| TEXAS INSTRUMENTS INCORPORATED
| Standard Linear and Logic Group
| IBIS Model of SN74ALVC164245
| 16-BIT 2.5-V TO 3.3-V/3.3-V TO 5-V LEVEL-SHIFTING TRANSCEIVER WITH
| 3-STATE OUTPUTS
| This file contains package information for the following:
|  TSSOP 48-pin (DGG) package as [Component] ALVC164245_DGG
|  SSOP 48-pin (DL) package as [Component] ALVC164245_DL
|  VFBGA 48-pin (GQL) package as [Component] ALVC164245_GQL
|  VFBGA 48-pin (ZQL) package as [Component] ALVC164245_ZQL
| This device can be powered at the following Vccs:
|  2.5 volt Vcc
|  3.3 volt Vcc
|  5.0 volt Vcc
| This file provides unique models under the [Model Selector] for each Vcc.
| For operation at a specific Vcc, select the appropriate model after each
| [Model Selector] keyword.
[IBIS Ver]   3.2
[Comment char]  |_char
[File Name]   sn74alvc164245.ibs
[File Rev]   1.1 | b_die
[Date]   September 14, 2004
[Source]   Data created from TI-SPICE simulations at TI-SLL.
[Notes]   The following is an IBIS list for the ALVC164245.
   Please contact sllibis@ti.com with questions and
   comments concerning SLL IBIS models.
   This IBIS model is created from a BA (back annotated
   netlist)
   - FILE REV HISTORY
   - 1.1 Release IBIS file on 09/29/04
   - Power clamp data has been deleted from DIR and NOE models
   since there is no power clamp diode for those inputs.
[Disclaimer] Property of Texas Instruments Incorporated.  Unauthorized
   reproduction and/or distribution is strictly prohibited.
   This product is protected under copyright law.
   Created  2004, (C) Copyright  2004, Texas Instruments
   Incorporated, All Rights Reserved
   UNLESS THERE IS A SIGNED, WRITTEN AGREEMENT TO THE
   CONTRARY, TEXAS INSTRUMENTS (TI) IS PROVIDING THE IBIS
   MODELS  AND WITHOUT ANY WARRANTY, EXPRESSED OR
   IMPLIED.  TI assumes no liability for:
   1) the accuracy of the IBIS models provided to your
   company;
   2) the proper functioning of these IBIS Models in your
   design or for any resulting applications; or
   3) infringement of patents, copyrights or intellectual
   property rights resulting from your use of these IBIS
   models.
   TI provides IBIS Models as a service to our customers.
   You and your company shall not distribute, sell or give
   these models to anyone else without prior written
   permission from TI.
   TI reserves the right to make changes to our products or
   to discontinue any semiconductor product or service
   without notice, and advises our customers to obtain the
   latest version of relevant information to verify, before
   placing orders, that the information being relied on is
   current.
   Please be aware that your receipt and use of the IBIS
   information provided shall serve as acceptance of these
   terms and conditions.  If you do not accept these terms,
   you should return or destroy the IBIS models and any
   other accompanying information immediately.
| Component ALVC164245_DGG 48-pin TSSOP
[Component]   ALVC164245_DGG
[Manufacturer]   Texas Instruments, Inc.
[Package]
|   typ   min   max
R_pkg   4.400e-02   3.800e-02   5.100e-02
L_pkg   3.019e-09   2.486e-09   4.099e-09
C_pkg   5.070e-13   3.340e-13   8.090e-13
[Pin]   signal_name   model_name   R_pin   L_pin   C_pin
1   1DIR   ALVC164245_DIR   4.100e-02   4.017e-09   7.590e-13
2   1B1   ALVC164245_BIO   4.200e-02   3.737e-09   7.920e-13
3   1B2   ALVC164245_BIO   4.200e-02   3.480e-09   6.610e-13
4   GND   GND   3.800e-02   3.131e-09   5.750e-13
5   1B3   ALVC164245_BIO   4.700e-02   3.122e-09   5.660e-13
6   1B4   ALVC164245_BIO   4.300e-02   2.948e-09   5.040e-13
7   VCCB   POWER   4.500e-02   2.845e-09   3.970e-13
8   1B5   ALVC164245_BIO   4.900e-02   2.835e-09   3.940e-13
9   1B6   ALVC164245_BIO   4.800e-02   2.715e-09   3.780e-13
10   GND   GND   5.000e-02   2.664e-09   3.630e-13
11   1B7   ALVC164245_BIO   5.000e-02   2.585e-09   3.480e-13
12   1B8   ALVC164245_BIO   4.900e-02   2.550e-09   3.370e-13
13   2B1   ALVC164245_BIO   4.900e-02   2.541e-09   3.360e-13
14   2B2   ALVC164245_BIO   5.000e-02   2.574e-09   3.480e-13
15   GND   GND   4.900e-02   2.618e-09   3.590e-13
16   2B3   ALVC164245_BIO   4.600e-02   2.671e-09   3.750e-13
17   2B4   ALVC164245_BIO   4.500e-02   2.754e-09   3.890e-13
18   VCCB   POWER   4.400e-02   2.823e-09   4.500e-13
19   2B5   ALVC164245_BIO   4.200e-02   2.968e-09   5.030e-13
20   2B6   ALVC164245_BIO   5.100e-02   3.108e-09   5.350e-13
21   GND   GND   4.200e-02   3.175e-09   5.870e-13
22   2B7   ALVC164245_BIO   4.100e-02   3.449e-09   6.780e-13
23   2B8   ALVC164245_BIO   4.400e-02   3.766e-09   8.040e-13
24   2DIR   ALVC164245_DIR   4.300e-02   4.065e-09   7.610e-13
25   2NOE   ALVC164245_NOE   4.100e-02   3.994e-09   7.570e-13
26   2A8   ALVC164245_AIO   3.900e-02   3.649e-09   7.890e-13
27   2A7   ALVC164245_AIO   3.800e-02   3.362e-09   6.600e-13
28   GND   GND   3.800e-02   3.082e-09   5.740e-13
29   2A6   ALVC164245_AIO   4.400e-02   2.990e-09   5.220e-13
30   2A5   ALVC164245_AIO   4.100e-02   2.917e-09   4.950e-13
31   VCCA   POWER   4.300e-02   2.820e-09   4.480e-13
32   2A4   ALVC164245_AIO   4.300e-02   2.699e-09   3.850e-13
33   2A3   ALVC164245_AIO   4.500e-02   2.628e-09   3.720e-13
34   GND   GND   4.600e-02   2.556e-09   3.560e-13
35   2A2   ALVC164245_AIO   4.600e-02   2.495e-09   3.440e-13
36   2A1   ALVC164245_AIO   4.700e-02   2.487e-09   3.340e-13
37   1A8   ALVC164245_AIO   4.700e-02   2.490e-09   3.350e-13
38   1A7   ALVC164245_AIO   4.600e-02   2.486e-09   3.430e-13
39   GND   GND   4.500e-02   2.566e-09   3.560e-13
40   1A6   ALVC164245_AIO   4.400e-02   2.639e-09   3.740e-13
41   1A5   ALVC164245_AIO   4.300e-02   2.701e-09   3.860e-13
42   VCCA   POWER   4.300e-02   2.817e-09   4.500e-13
43   1A4   ALVC164245_AIO   4.100e-02   2.935e-09   5.010e-13
44   1A3   ALVC164245_AIO   4.700e-02   3.035e-09   5.290e-13
45   GND   GND   4.300e-02   3.171e-09   5.890e-13
46   1A2   ALVC164245_AIO   4.000e-02   3.415e-09   6.820e-13
47   1A1   ALVC164245_AIO   4.300e-02   3.741e-09   8.090e-13
48   1NOE   ALVC164245_NOE   4.400e-02   4.099e-09   7.640e-13
| Component ALVC164245_DL 48-pin SSOP
[Component]   ALVC164245_DL
[Manufacturer]   Texas Instruments, Inc.
[Package]
|   typ   min   max
R_pkg   4.800e-02   3.800e-02   5.300e-02
L_pkg   6.046e-09   5.084e-09   7.968e-09
C_pkg   8.130e-13   5.690e-13   1.157e-12
[Pin]   signal_name   model_name   R_pin   L_pin   C_pin
1   1DIR   ALVC164245_DIR   4.600e-02   7.968e-09   1.017e-12
2   1B1   ALVC164245_BIO   4.400e-02   7.299e-09   1.157e-12
3   1B2   ALVC164245_BIO   4.300e-02   6.765e-09   1.058e-12
4   GND   GND   4.100e-02   6.269e-09   9.330e-13
5   1B3   ALVC164245_BIO   3.800e-02   5.856e-09   8.290e-13
6   1B4   ALVC164245_BIO   4.600e-02   5.802e-09   7.900e-13
7   VCCB   POWER   5.000e-02   5.656e-09   7.380e-13
8   1B5   ALVC164245_BIO   5.300e-02   5.500e-09   6.430e-13
9   1B6   ALVC164245_BIO   5.200e-02   5.304e-09   6.060e-13
10   GND   GND   5.300e-02   5.189e-09   5.830e-13
11   1B7   ALVC164245_BIO   5.100e-02   5.084e-09   5.690e-13
12   1B8   ALVC164245_BIO   5.300e-02   5.862e-09   8.330e-13
13   2B1   ALVC164245_BIO   5.300e-02   5.862e-09   8.330e-13
14   2B2   ALVC164245_BIO   5.100e-02   5.084e-09   5.690e-13
15   GND   GND   5.300e-02   5.189e-09   5.830e-13
16   2B3   ALVC164245_BIO   5.200e-02   5.304e-09   6.060e-13
17   2B4   ALVC164245_BIO   5.300e-02   5.500e-09   6.430e-13
18   VCCB   POWER   5.000e-02   5.656e-09   7.380e-13
19   2B5   ALVC164245_BIO   4.600e-02   5.802e-09   7.900e-13
20   2B6   ALVC164245_BIO   3.800e-02   5.856e-09   8.290e-13
21   GND   GND   4.100e-02   6.269e-09   9.330e-13
22   2B7   ALVC164245_BIO   4.300e-02   6.765e-09   1.058e-12
23   2B8   ALVC164245_BIO   4.400e-02   7.299e-09   1.157e-12
24   2DIR   ALVC164245_DIR   4.600e-02   7.968e-09   1.017e-12
25   2NOE   ALVC164245_NOE   4.600e-02   7.968e-09   1.017e-12
26   2A8   ALVC164245_AIO   4.400e-02   7.299e-09   1.157e-12
27   2A7   ALVC164245_AIO   4.300e-02   6.765e-09   1.058e-12
28   GND   GND   4.100e-02   6.269e-09   9.330e-13
29   2A6   ALVC164245_AIO   3.800e-02   5.856e-09   8.290e-13
30   2A5   ALVC164245_AIO   4.600e-02   5.802e-09   7.900e-13
31   VCCA   POWER   5.000e-02   5.656e-09   7.380e-13
32   2A4   ALVC164245_AIO   5.300e-02   5.500e-09   6.430e-13
33   2A3   ALVC164245_AIO   5.200e-02   5.304e-09   6.060e-13
34   GND   GND   5.300e-02   5.189e-09   5.830e-13
35   2A2   ALVC164245_AIO   5.100e-02   5.084e-09   5.690e-13
36   2A1   ALVC164245_AIO   5.300e-02   5.862e-09   8.330e-13
37   1A8   ALVC164245_AIO   5.300e-02   5.862e-09   8.330e-13
38   1A7   ALVC164245_AIO   5.100e-02   5.084e-09   5.690e-13
39   GND   GND   5.300e-02   5.189e-09   5.830e-13
40   1A6   ALVC164245_AIO   5.200e-02   5.304e-09   6.060e-13
41   1A5   ALVC164245_AIO   5.300e-02   5.500e-09   6.430e-13
42   VCCA   POWER   5.000e-02   5.656e-09   7.380e-13
43   1A4   ALVC164245_AIO   4.600e-02   5.802e-09   7.900e-13
44   1A3   ALVC164245_AIO   3.800e-02   5.856e-09   8.290e-13
45   GND   GND   4.100e-02   6.269e-09   9.330e-13
46   1A2   ALVC164245_AIO   4.300e-02   6.765e-09   1.058e-12
47   1A1   ALVC164245_AIO   4.400e-02   7.299e-09   1.157e-12
48   1NOE   ALVC164245_NOE   4.600e-02   7.967e-09   1.017e-12
| Component ALVC164245_GQL 48-pin VFBGA
[Component]   ALVC164245_GQL
[Manufacturer]   Texas Instruments, Inc.
[Package]
|   typ   min   max
R_pkg   7.900e-02   4.500e-02   9.400e-02
L_pkg   2.264e-09   1.398e-09   2.722e-09
C_pkg   3.060e-13   1.170e-13   4.040e-13
[Pin]   signal_name   model_name   R_pin   L_pin   C_pin
A1   1DIR   ALVC164245_DIR   5.10E-02   1.53E-09   2.10E-13
B2   1B1   ALVC164245_BIO   7.30E-02   2.57E-09   3.12E-13
B1   1B2   ALVC164245_BIO   7.10E-02   1.84E-09   2.32E-13
B3   GND   GND   9.40E-02   2.72E-09   3.83E-13
C2   1B3   ALVC164245_BIO   8.90E-02   2.53E-09   3.50E-13
C1   1B4   ALVC164245_BIO   7.10E-02   1.83E-09   2.31E-13
C3   VCCB   POWER   9.40E-02   2.72E-09   3.92E-13
D2   1B5   ALVC164245_BIO   9.00E-02   2.55E-09   3.52E-13
D1   1B6   ALVC164245_BIO   7.20E-02   1.85E-09   2.44E-13
D3   GND   GND   9.40E-02   2.72E-09   4.03E-13
E2   1B7   ALVC164245_BIO   8.90E-02   2.54E-09   3.51E-13
E1   1B8   ALVC164245_BIO   7.20E-02   1.85E-09   2.27E-13
F1   2B1   ALVC164245_BIO   7.20E-02   1.85E-09   2.27E-13
F2   2B2   ALVC164245_BIO   8.90E-02   2.54E-09   3.51E-13
G3   GND   GND   9.40E-02   2.72E-09   4.04E-13
G1   2B3   ALVC164245_BIO   7.20E-02   1.85E-09   2.44E-13
G2   2B4   ALVC164245_BIO   9.00E-02   2.55E-09   3.52E-13
H3   VCCB   POWER   9.40E-02   2.72E-09   3.92E-13
H1   2B5   ALVC164245_BIO   7.00E-02   1.83E-09   2.31E-13
H2   2B6   ALVC164245_BIO   8.80E-02   2.52E-09   3.50E-13
J3   GND   GND   9.30E-02   2.71E-09   3.82E-13
J1   2B7   ALVC164245_BIO   7.10E-02   1.85E-09   2.33E-13
J2   2B8   ALVC164245_BIO   5.60E-02   2.61E-09   3.90E-13
K1   2DIR   ALVC164245_DIR   4.50E-02   1.40E-09   1.17E-13
K6   2NOE   ALVC164245_NOE   4.50E-02   1.51E-09   1.93E-13
J5   2A8   ALVC164245_AIO   5.50E-02   2.49E-09   3.13E-13
J6   2A7   ALVC164245_AIO   7.00E-02   1.82E-09   2.30E-13
J4   GND   GND   9.30E-02   2.70E-09   3.82E-13
H5   2A6   ALVC164245_AIO   8.90E-02   2.53E-09   3.50E-13
H6   2A5   ALVC164245_AIO   7.10E-02   1.83E-09   2.30E-13
H4   VCCA   POWER   9.40E-02   2.72E-09   3.91E-13
G5   2A4   ALVC164245_AIO   9.00E-02   2.55E-09   3.52E-13
G6   2A3   ALVC164245_AIO   7.20E-02   1.85E-09   2.44E-13
G4   GND   GND   9.40E-02   2.72E-09   4.04E-13
F5   2A2   ALVC164245_AIO   8.80E-02   2.51E-09   3.49E-13
F6   2A1   ALVC164245_AIO   7.20E-02   1.85E-09   2.27E-13
E6   1A8   ALVC164245_AIO   7.10E-02   1.85E-09   2.27E-13
E5   1A7   ALVC164245_AIO   8.90E-02   2.53E-09   3.50E-13
D4   GND   GND   9.40E-02   2.72E-09   4.03E-13
D6   1A6   ALVC164245_AIO   7.20E-02   1.85E-09   2.43E-13
D5   1A5   ALVC164245_AIO   8.90E-02   2.55E-09   3.52E-13
C4   VCCA   POWER   9.40E-02   2.72E-09   3.91E-13
C6   1A4   ALVC164245_AIO   7.10E-02   1.83E-09   2.30E-13
C5   1A3   ALVC164245_AIO   8.90E-02   2.54E-09   3.50E-13
B4   GND   GND   9.30E-02   2.71E-09   3.82E-13
B6   1A2   ALVC164245_AIO   7.10E-02   1.83E-09   2.27E-13
B5   1A1   ALVC164245_AIO   7.30E-02   2.69E-09   3.80E-13
A6   1NOE   ALVC164245_NOE   5.10E-02   1.42E-09   1.33E-13
| Component ALVC164245_ZQL 48-pin VFBGA
[Component]   ALVC164245_ZQL
[Manufacturer]   Texas Instruments, Inc.
[Package]
|   typ   min   max
R_pkg   7.900e-02   4.500e-02   9.400e-02
L_pkg   2.264e-09   1.398e-09   2.722e-09
C_pkg   3.060e-13   1.170e-13   4.040e-13
[Pin]   signal_name   model_name   R_pin   L_pin   C_pin
A1   1DIR   ALVC164245_DIR   5.10E-02   1.53E-09   2.10E-13
B2   1B1   ALVC164245_BIO   7.30E-02   2.57E-09   3.12E-13
B1   1B2   ALVC164245_BIO   7.10E-02   1.84E-09   2.32E-13
B3   GND   GND   9.40E-02   2.72E-09   3.83E-13
C2   1B3   ALVC164245_BIO   8.90E-02   2.53E-09   3.50E-13
C1   1B4   ALVC164245_BIO   7.10E-02   1.83E-09   2.31E-13
C3   VCCB   POWER   9.40E-02   2.72E-09   3.92E-13
D2   1B5   ALVC164245_BIO   9.00E-02   2.55E-09   3.52E-13
D1   1B6   ALVC164245_BIO   7.20E-02   1.85E-09   2.44E-13
D3   GND   GND   9.40E-02   2.72E-09   4.03E-13
E2   1B7   ALVC164245_BIO   8.90E-02   2.54E-09   3.51E-13
E1   1B8   ALVC164245_BIO   7.20E-02   1.85E-09   2.27E-13
F1   2B1   ALVC164245_BIO   7.20E-02   1.85E-09   2.27E-13
F2   2B2   ALVC164245_BIO   8.90E-02   2.54E-09   3.51E-13
G3   GND   GND   9.40E-02   2.72E-09   4.04E-13
G1   2B3   ALVC164245_BIO   7.20E-02   1.85E-09   2.44E-13
G2   2B4   ALVC164245_BIO   9.00E-02   2.55E-09   3.52E-13
H3   VCCB   POWER   9.40E-02   2.72E-09   3.92E-13
H1   2B5   ALVC164245_BIO   7.00E-02   1.83E-09   2.31E-13
H2   2B6   ALVC164245_BIO   8.80E-02   2.52E-09   3.50E-13
J3   GND   GND   9.30E-02   2.71E-09   3.82E-13
J1   2B7   ALVC164245_BIO   7.10E-02   1.85E-09   2.33E-13
J2   2B8   ALVC164245_BIO   5.60E-02   2.61E-09   3.90E-13
K1   2DIR   ALVC164245_DIR   4.50E-02   1.40E-09   1.17E-13
K6   2NOE   ALVC164245_NOE   4.50E-02   1.51E-09   1.93E-13
J5   2A8   ALVC164245_AIO   5.50E-02   2.49E-09   3.13E-13
J6   2A7   ALVC164245_AIO   7.00E-02   1.82E-09   2.30E-13
J4   GND   GND   9.30E-02   2.70E-09   3.82E-13
H5   2A6   ALVC164245_AIO   8.90E-02   2.53E-09   3.50E-13
H6   2A5   ALVC164245_AIO   7.10E-02   1.83E-09   2.30E-13
H4   VCCA   POWER   9.40E-02   2.72E-09   3.91E-13
G5   2A4   ALVC164245_AIO   9.00E-02   2.55E-09   3.52E-13
G6   2A3   ALVC164245_AIO   7.20E-02   1.85E-09   2.44E-13
G4   GND   GND   9.40E-02   2.72E-09   4.04E-13
F5   2A2   ALVC164245_AIO   8.80E-02   2.51E-09   3.49E-13
F6   2A1   ALVC164245_AIO   7.20E-02   1.85E-09   2.27E-13
E6   1A8   ALVC164245_AIO   7.10E-02   1.85E-09   2.27E-13
E5   1A7   ALVC164245_AIO   8.90E-02   2.53E-09   3.50E-13
D4   GND   GND   9.40E-02   2.72E-09   4.03E-13
D6   1A6   ALVC164245_AIO   7.20E-02   1.85E-09   2.43E-13
D5   1A5   ALVC164245_AIO   8.90E-02   2.55E-09   3.52E-13
C4   VCCA   POWER   9.40E-02   2.72E-09   3.91E-13
C6   1A4   ALVC164245_AIO   7.10E-02   1.83E-09   2.30E-13
C5   1A3   ALVC164245_AIO   8.90E-02   2.54E-09   3.50E-13
B4   GND   GND   9.30E-02   2.71E-09   3.82E-13
B6   1A2   ALVC164245_AIO   7.10E-02   1.83E-09   2.27E-13
B5   1A1   ALVC164245_AIO   7.30E-02   2.69E-09   3.80E-13
A6   1NOE   ALVC164245_NOE   5.10E-02   1.42E-09   1.33E-13
| Model ALVC164245_DIR
[Model Selector]   ALVC164245_DIR
ALVC164245_DIR_25   2.5 volt Vcc
ALVC164245_DIR_33   3.3 volt Vcc
ALVC164245_DIR_50   5 volt Vcc
| Model ALVC164245_NOE
[Model Selector]   ALVC164245_NOE
ALVC164245_NOE_25   2.5 volt Vcc
ALVC164245_NOE_33   3.3 volt Vcc
ALVC164245_NOE_50   5 volt Vcc
| Model ALVC164245_AIO
[Model Selector]   ALVC164245_AIO
ALVC164245_AIO_25   2.5 volt Vcc
ALVC164245_AIO_33   3.3 volt Vcc
| Model ALVC164245_BIO
[Model Selector]   ALVC164245_BIO
ALVC164245_BIO_33   3.3 volt Vcc
ALVC164245_BIO_50   5 volt Vcc
| Models and submodels in the file (10): ALVC164245_DIR_25 (Input), ALVC164245_DIR_33 (Input), ALVC164245_DIR_50 (Input), ALVC164245_NOE_25 (Input), ALVC164245_NOE_33 (Input), ALVC164245_NOE_50 (Input), ALVC164245_AIO_25 (I/O), ALVC164245_AIO_33 (I/O), ALVC164245_BIO_33 (I/O), ALVC164245_BIO_50 (I/O)
